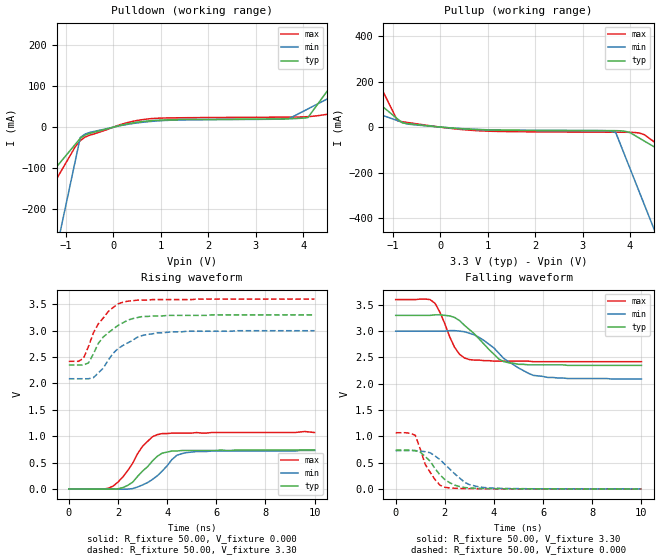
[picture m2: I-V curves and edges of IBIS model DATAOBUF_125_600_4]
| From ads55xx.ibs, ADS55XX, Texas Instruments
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|   Model DATAOBUF_125_600_4
[Model]   DATAOBUF_125_600_4
Model_type   Output
Polarity   Non-Inverting
Vmeas =   1.65V
C_comp   3.00pF   3.00pF   3.00pF
[Temperature Range]   50.00   0.10k   -20.00
[Voltage Range]   3.30V   3.00V   3.60V
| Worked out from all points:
|   slope of the pulldown table from 0 to 0.495 V, typ, clamps not added: 41.7 ohm
|   slope of the pullup table from 0 to 0.495 V, typ, clamps not added: 61.3 ohm
|   rising waveform, R_fixture 50.00, V_fixture 0.000: 20-80 % time 905ps typ, 973ps min, 934ps max; typ from 0 V to 0.74 V
|   rising waveform, R_fixture 50.00, V_fixture 3.30: 20-80 % time 1.06ns typ, 1.23ns min, 850ps max; typ from 2.35 V to 3.3 V
|   falling waveform, R_fixture 50.00, V_fixture 3.30: 20-80 % time 1.24ns typ, 1.51ns min, 657ps max; typ from 3.3 V to 2.35 V
|   falling waveform, R_fixture 50.00, V_fixture 0.000: 20-80 % time 842ps typ, 1.03ns min, 624ps max; typ from 0.74 V to 0.001 V
[Pulldown]
| voltage   I(typ)   I(min)   I(max)
-3.3V     -388.8mA   -1.437A    -543.2mA
-2.3V     -249.7mA   -893.7mA   -344.6mA
-1.9V     -194.1mA   -676.6mA   -265.1mA
-1.7V     -166.3mA   -568.1mA   -225.4mA
-1.5V     -138.4mA   -459.5mA   -185.7mA
-1V       -68.88mA   -188.1mA   -86.41mA
-700mV    -27.15mA   -25.27mA   -33.1mA
300mV     8.13mA     6.82mA     11.17mA
3.7V      20.36mA    20.56mA    24.45mA
4.1V      23.23mA    44.32mA    25.53mA
5.5V      245.4mA    127.5mA    48.36mA
6.6V      420mA      192.8mA    67.33mA
[Pullup]
| voltage   I(typ)   I(min)   I(max)
-3.3V     450.4mA    205.4mA    1.037A
-3.1V     415.8mA    190.6mA    952.8mA
-1.9V     208.6mA    102.2mA    448mA
-900mV    35.88mA    28.51mA    27.29mA
-800mV    18.61mA    21.14mA    23.8mA
800mV     -10.96mA   -10.11mA   -15.83mA
3.6V      -15.39mA   -17.89mA   -22.33mA
3.7V      -15.53mA   -24.49mA   -22.4mA
4V        -24.16mA   -182.7mA   -22.86mA
4.2V      -48.82mA   -288.1mA   -26.02mA
4.5V      -85.81mA   -446.3mA   -63.44mA
6.6V      -344.7mA   -1.554A    -383.1mA
[Ramp]
| variable   typ   min   max
dV/dt_r   0.44/0.87n   0.44/1.00n   0.64/0.95n
dV/dt_f   0.57/1.18n   0.54/1.48n   0.71/0.64n
R_load = 50.00
[Rising Waveform]
R_fixture = 50.00
V_fixture = 0.000
V_fixture_min = 0.000
V_fixture_max = 0.000
| time   V(typ)   V(min)   V(max)
0s        13.98nV    17.2nV     26.84nV
1.4ns     -1.58mV    -2.21mV    -1.71mV
1.8ns     -2.79mV    -1.84mV    54.94mV
2.2ns     27.21mV    -3.22mV    230mV
2.6ns     130mV      7.64mV     490mV
3ns       340mV      76.79mV    810mV
3.6ns     620mV      250mV      1.03V
4.4ns     720mV      640mV      1.06V
4.8ns     730mV      690mV      1.06V
10ns      740mV      730mV      1.07V
[Rising Waveform]
R_fixture = 50.00
V_fixture = 3.30
V_fixture_min = 3.00
V_fixture_max = 3.60
| time   V(typ)   V(min)   V(max)
0s        2.35V      2.09V      2.42V
600ps     2.35V      2.09V      2.48V
800ps     2.39V      2.09V      2.7V
1ns       2.56V      2.11V      2.96V
1.4ns     2.88V      2.29V      3.24V
1.8ns     3.03V      2.57V      3.44V
2.2ns     3.15V      2.72V      3.54V
2.8ns     3.25V      2.88V      3.58V
3.6ns     3.28V      2.96V      3.59V
10ns      3.3V       3V         3.6V
[Falling Waveform]
R_fixture = 50.00
V_fixture = 3.30
V_fixture_min = 3.00
V_fixture_max = 3.60
| time   V(typ)   V(min)   V(max)
0s        3.3V       3V         3.6V
1.2ns     3.3V       3V         3.61V
1.6ns     3.31V      3V         3.53V
2.4ns     3.26V      3.01V      2.69V
2.6ns     3.2V       3V         2.56V
3ns       3.03V      2.96V      2.46V
3.6ns     2.75V      2.82V      2.44V
4.2ns     2.47V      2.58V      2.43V
5.6ns     2.36V      2.16V      2.42V
10ns      2.35V      2.09V      2.42V
[Falling Waveform]
R_fixture = 50.00
V_fixture = 0.000
V_fixture_min = 0.000
V_fixture_max = 0.000
| time   V(typ)   V(min)   V(max)
0s        740mV      730mV      1.07V
800ps     730mV      730mV      1.02V
1.2ns     620mV      710mV      470mV
1.6ns     390mV      630mV      180mV
1.8ns     270mV      560mV      73.81mV
2ns       180mV      470mV      33.8mV
2.4ns     74.64mV    290mV      15.18mV
2.8ns     28.76mV    130mV      8.92mV
3.4ns     13.77mV    40.06mV    6.03mV
10ns      1.27mV     1.61mV     1.05mV
